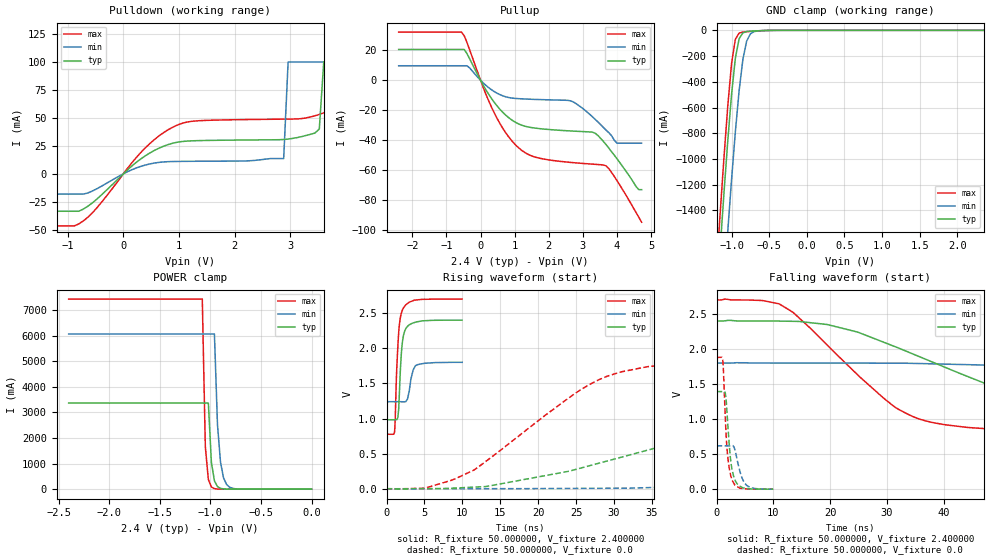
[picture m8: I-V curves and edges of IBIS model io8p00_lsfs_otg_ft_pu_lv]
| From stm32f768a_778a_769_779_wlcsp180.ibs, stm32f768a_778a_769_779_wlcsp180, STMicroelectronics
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|   Model io8p00_lsfs_otg_ft_pu_lv
[Model]  io8p00_lsfs_otg_ft_pu_lv
Model_type I/O
Polarity   Non-Inverting
Enable   Active-Low
Vinl =   0.720000V
Vinh =   1.680000V
Vmeas =  1.200000V
Cref =   50.000000pF
Rref =   100.000000M
Vref =   0.0V
C_comp   7.971100pF   7.737700pF   8.264100pF
[Temperature Range]   25.000000   0.125000k   -40.000000
[Pullup Reference]   2.400000V   1.800000V   2.700000V
[Pulldown Reference]   0.0V   0.0V   0.0V
[POWER Clamp Reference]   2.400000V   1.800000V   2.700000V
[GND Clamp Reference]   0.0V   0.0V   0.0V
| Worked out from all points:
|   slope of the pulldown table from 0 to 0.36 V, typ, clamps not added: 24.1 ohm
|   slope of the pullup table from 0 to 0.36 V, typ, clamps not added: 26.8 ohm
|   GND clamp passes 1 mA (typ) near -0.52 V on its own axis
|   POWER clamp passes 1 mA (typ) near -0.81 V on its own axis
|   rising waveform, R_fixture 50.000000, V_fixture 2.400000: 20-80 % time 475ps typ, 591ps min, 487ps max; typ from 0.983 V to 2.4 V
|   rising waveform, R_fixture 50.000000, V_fixture 0.0: 20-80 % time 30.9ns typ, 82.1ns min, 14.2ns max; typ from 0.001 V to 1.39 V
|   falling waveform, R_fixture 50.000000, V_fixture 2.400000: 20-80 % time 28.6ns typ, 71.1ns min, 15.4ns max; typ from 2.4 V to 0.983 V
|   falling waveform, R_fixture 50.000000, V_fixture 0.0: 20-80 % time 911ps typ, 1.27ns min, 795ps max; typ from 1.39 V to 0.001 V
[Pulldown]
|Voltage   I(typ)   I(min)   I(max)
-2.4V     -33.44mA   -18.11mA   -46.51mA
-800mV    -33.44mA   -18.11mA   -44.78mA
1.04V     28.81mA    11.14mA    44.91mA
2.88V     30.7mA     13.62mA    48.89mA
2.96V     31.1mA     100mA      48.94mA
3.52V     40mA       100mA      53.06mA
3.6V      100mA      100mA      54.54mA
3.92V     100mA      100mA      60mA
4V        100mA      100mA      100mA
4.4V      100mA      100mA      100mA
4.48V     100mA      100mA      1A
4.8V      100mA      100mA      1A
[Pullup]
|Voltage   I(typ)   I(min)   I(max)
-2.4V     20.55mA    9.685mA    32.15mA
-560mV    20.55mA    9.685mA    32.15mA
-400mV    17.86mA    9.685mA    25.31mA
320mV     -12.14mA   -6.322mA   -17.91mA
960mV     -27.18mA   -12mA      -41.54mA
1.52V     -31.65mA   -12.71mA   -50.67mA
2.64V     -33.82mA   -13.73mA   -54.81mA
3.28V     -34.63mA   -24.4mA    -55.96mA
3.68V     -43mA      -33.3mA    -57.12mA
4V        -52.4mA    -42mA      -67mA
4.56V     -71mA      -42mA      -88.3mA
4.72V     -73mA      -42mA      -94.7mA
[GND_clamp]
|Voltage   I(typ)   I(min)   I(max)
-2.4V     -9.766A    -9.942A    -9.572A
-1.2V     -2.124A    -2.851A    -1.855A
-1.15V    -1.682A    -2.408A    -1.408A
-1.1V     -1.256A    -1.975A    -979.8mA
-1.05V    -854.9mA   -1.556A    -584.5mA
-1V       -496.5mA   -1.158A    -257.5mA
-950mV    -217.7mA   -789.6mA   -69.52mA
-900mV    -65.57mA   -469.8mA   -21.5mA
-850mV    -19.64mA   -226.4mA   -13.56mA
-800mV    -9.753mA   -84.21mA   -10.47mA
-700mV    -4.923mA   -9.884mA   -5.807mA
2.35V     0A         0A         0A
[POWER_clamp]
|Voltage   I(typ)   I(min)   I(max)
-2.4V     3.365A     6.064A     7.43A
-1.08V    3.365A     6.064A     7.43A
-1.05V    3.365A     6.064A     1.669A
-1.02V    3.365A     6.064A     375.2mA
-990mV    1.047A     6.064A     84.45mA
-960mV    325.8mA    6.064A     19.12mA
-930mV    101.4mA    2.529A     4.431mA
-900mV    31.63mA    1.055A     1.12mA
-870mV    9.908mA    440.1mA    365.5uA
-840mV    3.145mA    183.6mA    185.6uA
-720mV    90.15uA    5.596mA    88.88uA
0V        0A         0A         0A
[Ramp]
| variable   typ   min   max
dV/dt_r  0.83577/30.94122n   0.36589/82.52513n   1.12831/14.18661n
dV/dt_f  0.85088/28.57770n   0.33156/72.85804n   1.15456/15.34611n
R_load = 50.000000
[Rising Waveform]
R_fixture= 50.000000
V_fixture= 2.400000
V_fixture_min= 1.800000
V_fixture_max= 2.700000
|time   V(typ)   V(min)   V(max)
0s        982.6mV    1.24V      775.9mV
1.061ns   982.4mV    1.24V      816.2mV
1.141ns   982.1mV    1.24V      976.3mV
1.341ns   984.4mV    1.24V      1.689V
1.562ns   1.088V     1.24V      2.159V
1.942ns   1.907V     1.239V     2.495V
2.182ns   2.153V     1.238V     2.564V
2.783ns   2.313V     1.283V     2.637V
3.824ns   2.371V     1.753V     2.686V
9.97ns    2.4V       1.8V       2.7V
[Rising Waveform]
R_fixture= 50.000000
V_fixture= 0.0
V_fixture_min= 0.0
V_fixture_max= 0.0
|time   V(typ)   V(min)   V(max)
0s        857.3uV    830.5uV    877.8uV
5.005ns   2.647mV    1.186mV    8.093mV
11.51ns   23.75mV    1.906mV    265.9mV
24.52ns   263.4mV    5.475mV    1.331V
29.03ns   393.8mV    7.796mV    1.599V
41.54ns   762.2mV    38.4mV     1.813V
62.06ns   1.213V     104mV      1.868V
81.08ns   1.34V      199mV      1.881V
165.2ns   1.392V     548.4mV    1.881V
249.2ns   1.393V     619.1mV    1.881V
[Falling Waveform]
R_fixture= 50.000000
V_fixture= 2.400000
V_fixture_min= 1.800000
V_fixture_max= 2.700000
|time   V(typ)   V(min)   V(max)
0s        2.4V       1.8V       2.7V
11.01ns   2.399V     1.8V       2.645V
19.52ns   2.35V      1.8V       2.056V
31.53ns   2.032V     1.798V     1.166V
36.54ns   1.865V     1.792V     981.9mV
44.04ns   1.615V     1.778V     883.1mV
61.56ns   1.206V     1.715V     816.9mV
87.09ns   1.051V     1.562V     787.5mV
160.2ns   990.1mV    1.293V     776.2mV
249.2ns   982.6mV    1.24V      775.9mV
[Falling Waveform]
R_fixture= 50.000000
V_fixture= 0.0
V_fixture_min= 0.0
V_fixture_max= 0.0
|time   V(typ)   V(min)   V(max)
0s        1.393V     619.1mV    1.881V
1.081ns   1.393V     619.1mV    1.852V
1.522ns   1.379V     619.1mV    1.075V
1.842ns   1.1V       618.7mV    584.6mV
2.402ns   480.3mV    620.3mV    230.7mV
2.763ns   270.8mV    623.3mV    126.1mV
3.504ns   90.84mV    469.1mV    45.34mV
4.484ns   26.13mV    162.3mV    11.53mV
5.285ns   12.2mV     56.71mV    4.954mV
9.97ns    857.3uV    830.5uV    877.8uV
